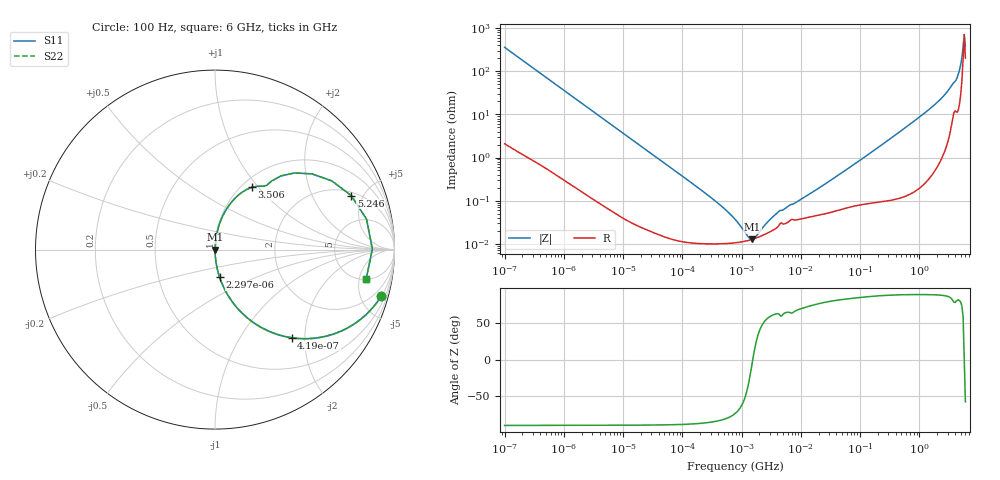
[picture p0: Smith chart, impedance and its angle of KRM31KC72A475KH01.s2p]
!Murata Part Number: KRM31KC72A475KH01
!These Parameters are Measured in Series Mode Connection
!Data Generated on Jan 08, 2026
!  o--ll--o
!Port1  Port2
!  o------o
!Operation Temp=25[degC], DC Bias Voltage=0[V]
!Freq. Start=100[Hz] Stop=6[GHz] 401[Steps]
# Hz S RI R 50
!Freq.(Hz) S11(Real) S11(Imag) S21(Real) S21(Imag) S12(Real) S12(Imag) S22(Real) S22(Imag)
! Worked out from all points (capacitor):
!   401 points, 100 Hz to 6 GHz, reference 50 ohm
!   read as one part in series: C = 4.43 uF near 109 Hz
!   lowest |Z| = 12.7 mohm at 1.516 MHz (marker M1)
!   series resonance near 1.545 MHz, so ESL is about 2.4 nH
!   S11 on the Smith chart (normalised r, x): 100 Hz: 1.04, -7.18; 419 Hz: 1.01, -1.72; 2.297 kHz: 1.00, -0.32; 3.506 GHz: 1.11, +0.92; 5.246 GHz: 2.24, +4.05; 6 GHz: 5.02, -6.31
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100  0.9267 -0.2577  0.0733 0.2577  0.0733 0.2577  0.9267 -0.2577
196  0.7703 -0.4174  0.2297 0.4174  0.2297 0.4174  0.7703 -0.4174
419  0.4269 -0.4909  0.5731 0.4909  0.5731 0.4909  0.4269 -0.4909
858  0.1536 -0.3565  0.8464 0.3565  0.8464 0.3565  0.1536 -0.3565
2008  0.0333 -0.175  0.9667 0.175  0.9667 0.175  0.0333 -0.175
2297  0.0259 -0.1544  0.9741 0.1544  0.9741 0.1544  0.0259 -0.1544
7036  0.00323 -0.0519  0.9968 0.0519  0.9968 0.0519  0.00323 -0.0519
40335  0.000245 -0.00917  0.9998 0.00917  0.9998 0.00917  0.000245 -0.00917
316350  0.0001 -0.00112  0.9999 0.00112  0.9999 0.00112  0.0001 -0.00112
774597  0.000105 -0.000356  0.9999 0.000356  0.9999 0.000356  0.000105 -0.000356
1267578  0.000118 -9.33e-05  0.9999 9.33e-05  0.9999 9.33e-05  0.000118 -9.33e-05
1516199  0.000127 -8.7e-06  0.9999 8.7e-06  0.9999 8.7e-06  0.000127 -8.7e-06
4060267  0.000245 0.000472  0.9998 -0.000472  0.9998 -0.000472  0.000245 0.000472
1.555665e7  0.00043 0.00149  0.9996 -0.00149  0.9996 -0.00149  0.00043 0.00149
3.124326e8  0.00169 0.0263  0.9983 -0.0263  0.9983 -0.0263  0.00169 0.0263
1.873145e9  0.0341 0.1674  0.9659 -0.1674  0.9659 -0.1674  0.0341 0.1674
2.679998e9  0.0853 0.256  0.9147 -0.256  0.9147 -0.256  0.0853 0.256
3.505958e9  0.2053 0.3469  0.7947 -0.3469  0.7947 -0.3469  0.2053 0.3469
4.586474e9  0.4443 0.4272  0.5557 -0.4272  0.5557 -0.4272  0.4443 0.4272
5.016141e9  0.65 0.3833  0.35 -0.3833  0.35 -0.3833  0.65 0.3833
5.245841e9  0.7592 0.3008  0.2408 -0.3008  0.2408 -0.3008  0.7592 0.3008
6e9  0.8417 -0.1658  0.1583 0.1658  0.1583 0.1658  0.8417 -0.1658
